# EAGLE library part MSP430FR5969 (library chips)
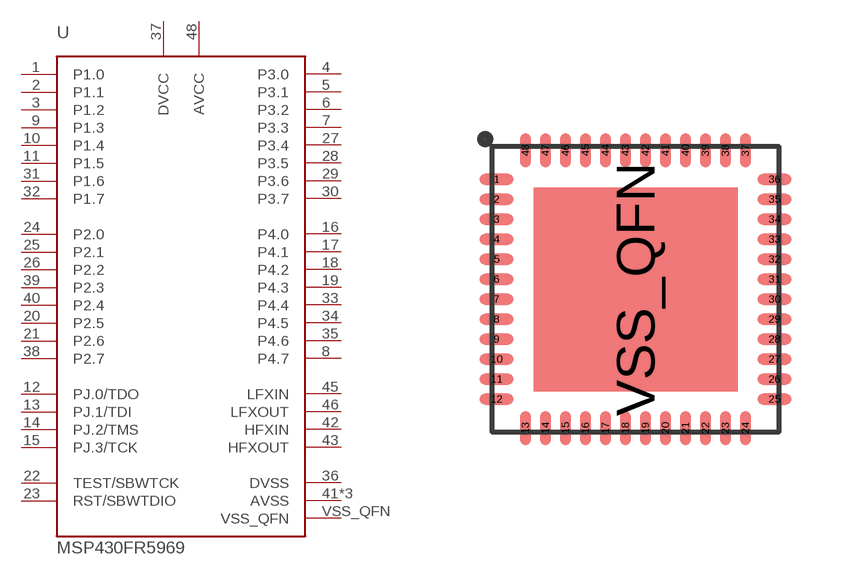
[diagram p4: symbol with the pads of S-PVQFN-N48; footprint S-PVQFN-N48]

Designator prefix U

## MSP430FR5969  [S-PVQFN-N48]
1  P1.0
2  P1.1
3  P1.2
4  P3.0
5  P3.1
6  P3.2
7  P3.3
8  P4.7
9  P1.3
10  P1.4
11  P1.5
12  PJ.0/TDO
13  PJ.1/TDI
14  PJ.2/TMS
15  PJ.3/TCK
16  P4.0
17  P4.1
18  P4.2
19  P4.3
20  P2.5
21  P2.6
22  TEST/SBWTCK
23  RST/SBWTDIO
24  P2.0
25  P2.1
26  P2.2
27  P3.4
28  P3.5
29  P3.6
30  P3.7
31  P1.6
32  P1.7
33  P4.4
34  P4.5
35  P4.6
36  DVSS
37  DVCC
38  P2.7
39  P2.3
40  P2.4
41  AVSS
42  HFXIN
43  HFXOUT
44  AVSS
45  LFXIN
46  LFXOUT
47  AVSS
48  AVCC
VSS_QFN  VSS_QFN

## Footprint S-PVQFN-N48 (pad centres in mm)
TI RGZ Package
smd 0.85 x 0.28: 1 -3.475,2.75; 2 -3.475,2.25; 3 -3.475,1.75; 4 -3.475,1.25; 5 -3.475,0.75; 6 -3.475,0.25; 7 -3.475,-0.25; 8 -3.475,-0.75; 9 -3.475,-1.25; 10 -3.475,-1.75; 11 -3.475,-2.25; 12 -3.475,-2.75; 25 3.475,-2.75; 26 3.475,-2.25; 27 3.475,-1.75; 28 3.475,-1.25; 29 3.475,-0.75; 30 3.475,-0.25; 31 3.475,0.25; 32 3.475,0.75; 33 3.475,1.25; 34 3.475,1.75; 35 3.475,2.25; 36 3.475,2.75
smd 0.28 x 0.85: 13 -2.75,-3.475; 14 -2.25,-3.475; 15 -1.75,-3.475; 16 -1.25,-3.475; 17 -0.75,-3.475; 18 -0.25,-3.475; 19 0.25,-3.475; 20 0.75,-3.475; 21 1.25,-3.475; 22 1.75,-3.475; 23 2.25,-3.475; 24 2.75,-3.475; 37 2.75,3.475; 38 2.25,3.475; 39 1.75,3.475; 40 1.25,3.475; 41 0.75,3.475; 42 0.25,3.475; 43 -0.25,3.475; 44 -0.75,3.475; 45 -1.25,3.475; 46 -1.75,3.475; 47 -2.25,3.475; 48 -2.75,3.475
smd 5.1 x 5.1: VSS_QFN 0,0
